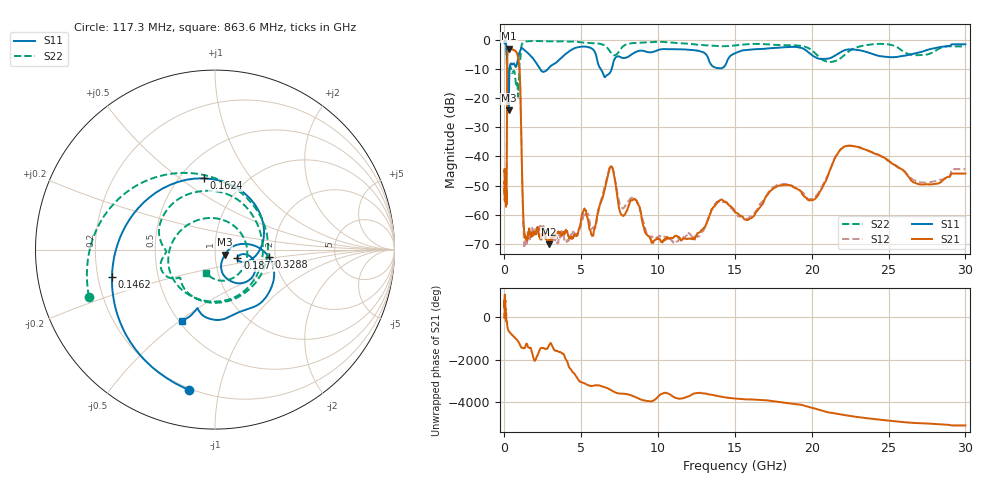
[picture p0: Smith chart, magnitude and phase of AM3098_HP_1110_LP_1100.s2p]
! Date/Time: Thu, Feb 28, 2019 8:47 AM
! Network Analyzer: Agilent Technologies E8364B Rev: A.07.50.67
! Sweep from 0.010 to 30.000 GHz, 1601 Points, Sweep Type: LOG
! Power Supply: 5.023 V, 0.002 A
# Hz S DB R 50
!freq MagS11 AngS11 MagS21 AngS21 MagS12 AngS12 MagS22 AngS22
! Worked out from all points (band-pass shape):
!   1601 points, 10 MHz to 30 GHz, reference 50 ohm
!   highest |S21| = -3.10 dB at 294.5 MHz (marker M1); lowest = -70.1 dB at 2.87 GHz (marker M2)
!   |S21| within 3 dB of the highest: 183.6 MHz to 887.3 MHz (703.7 MHz wide, 131 % of centre)
!   lowest |S11| = -24.1 dB at 266.5 MHz (marker M3), VSWR 1.13, Z = 55.7 - j3.18 ohm
!   |S11| at or under -10 dB: 169.6 MHz to 334.4 MHz (164.7 MHz wide, 65.4 % of centre); 2.323 GHz to 2.835 GHz (511.9 MHz wide, 19.9 % of centre); 6.256 GHz to 6.981 GHz (725 MHz wide, 11 % of centre)
!   |S22| runs from -19.6 to -0.5 dB; largest |S21 - S12| = 0.011
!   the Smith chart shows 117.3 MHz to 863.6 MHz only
!   S11 on the Smith chart (normalised r, x): 117.3 MHz: 0.19, -0.81; 146.2 MHz: 0.26, -0.12; 162.4 MHz: 0.65, +0.62; 187.7 MHz: 1.28, -0.12; 328.8 MHz: 1.84, -0.16; 863.6 MHz: 0.52, -0.51
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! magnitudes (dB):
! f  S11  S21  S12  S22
! 10 MHz  -0.4  -45.3  -44.6  -0.6
! 38.04 MHz  -0.3  -50.9  -51.0  -0.8
! 117.3 MHz  -2.0  -51.7  -53.2  -2.5
! 144.7 MHz  -4.3  -49.6  -49.6  -5.5
! 146.2 MHz  -4.5  -48.3  -48.2  -5.8
! 162.4 MHz  -7.9  -22.2  -22.2  -10.6
! 187.7 MHz  -17.5  -5.4  -5.4  -12.0
! 266.5 MHz  -24.1  -3.2  -3.1  -11.3
! 294.5 MHz  -15.5  -3.1  -3.0  -10.8
! 328.8 MHz  -10.4  -3.2  -3.1  -9.6
! 550.5 MHz  -8.3  -3.5  -3.4  -11.0
! 863.6 MHz  -7.2  -5.5  -5.5  -17.2
! 1.019 GHz  -3.9  -14.5  -14.5  -7.2
! 1.289 GHz  -3.6  -65.8  -70.4  -0.8
! 2.084 GHz  -8.1  -64.8  -67.0  -0.5
! 2.87 GHz  -9.8  -70.1  -67.1  -0.6
! 5.754 GHz  -3.3  -67.1  -64.3  -1.2
! 6.89 GHz  -11.1  -43.6  -43.5  -4.2
! 7.926 GHz  -6.2  -58.9  -56.5  -1.6
! 11.31 GHz  -3.3  -67.8  -69.0  -1.2
! 22.56 GHz  -3.3  -36.4  -36.3  -3.5
! 30 GHz  -1.6  -45.9  -44.4  -2.3
